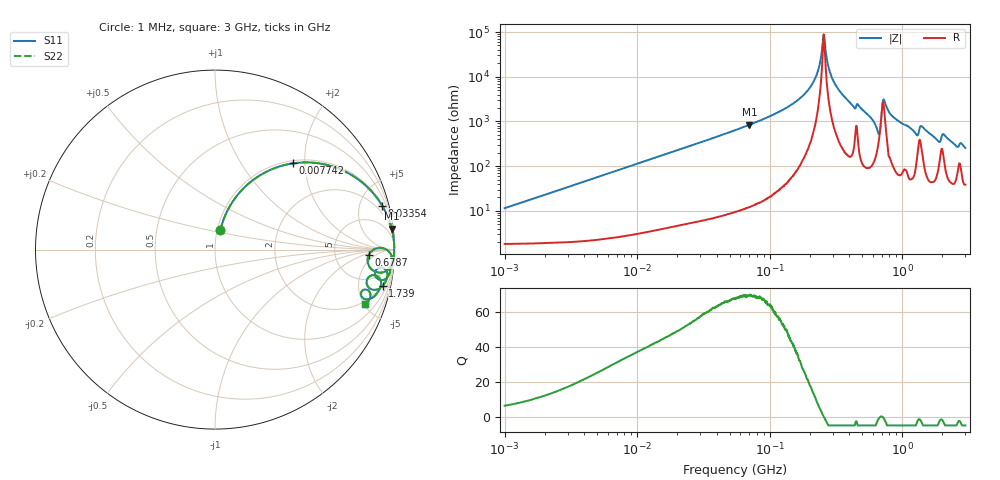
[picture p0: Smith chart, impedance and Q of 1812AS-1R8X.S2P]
!s-Parameter Generated by FASTRON Sdn. Bhd.
!FASTRON P/N : 1812AS-1R8X
!Keysight Technologies,E4991B,MY54100416,A.01.15
!Date created: Fri Oct 13 15:33:57 2023
!Version  : Rev00 Fri Oct 13 15:33:57 2023
!Data & Calibration Information:
!Freq	S11	S21	S12	S22
!PortZ  Port1:50+j0  Port2:50+j0
!When reading, reference impedance value at option line is always used.
! Remarks : This data is being provided solely for informational purposes.
# Hz S dB R 50
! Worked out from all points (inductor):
!   1601 points, 1 MHz to 3 GHz, reference 50 ohm
!   read as one part in series: L = 1.81 uH near 1.041 MHz
!   highest Q = 69.2 at 70.34 MHz (marker M1), where L = 1.9 uH
!   self-resonance near 255.8 MHz
!   S11 on the Smith chart (normalised r, x): 1 MHz: 1.04, +0.23; 7.742 MHz: 1.05, +1.74; 33.54 MHz: 1.13, +7.58; 678.7 MHz: 12, -3; 1.739 GHz: 1.90, -8.97; 3 GHz: 1.77, -5.06
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1000000  -19.00 74.5  -0.21 -6.4  -0.21 -6.4  -19.00 74.5
3804036  -8.21 64.4  -0.89 -22.8  -0.89 -22.8  -8.21 64.4
7741750  -3.77 47.9  -2.59 -40.4  -2.59 -40.4  -3.77 47.9
1.447069e7  -1.48 31.2  -5.70 -57.4  -5.70 -57.4  -1.48 31.2
3.354185e7  -0.33 14.7  -11.90 -74.3  -11.90 -74.3  -0.33 14.7
5.477226e7  -0.13 8.9  -16.19 -80.2  -16.19 -80.2  -0.13 8.9
7.034296e7  -0.08 6.8  -18.57 -82.4  -18.57 -82.4  -0.08 6.8
1.445978e8  -0.02 2.5  -27.34 -86.2  -27.34 -86.2  -0.02 2.5
2.083556e8  -0.01 0.9  -36.47 -85.4  -36.47 -85.4  -0.01 0.9
2.302869e8  -0.01 0.4  -42.20 -81.8  -42.20 -81.8  -0.01 0.4
2.570867e8  -0.01 -0.0  -58.66 12.9  -58.66 12.9  -0.01 -0.0
2.870054e8  -0.01 -0.5  -41.52 81.4  -41.52 81.4  -0.01 -0.5
3.301716e8  -0.01 -1.1  -34.35 84.8  -34.35 84.8  -0.01 -1.1
6.520712e8  -0.62 -7.9  -16.49 58.9  -16.49 58.9  -0.62 -7.9
6.787043e8  -1.34 -2.0  -16.66 11.8  -16.66 11.8  -1.34 -2.0
7.279565e8  -0.20 -1.3  -29.94 44.9  -29.94 44.9  -0.20 -1.3
7.925923e8  -0.07 -3.4  -24.41 80.8  -24.41 80.8  -0.07 -3.4
1.262285e9  -0.40 -10.1  -14.97 70.5  -14.97 70.5  -0.40 -10.1
1.409185e9  -0.36 -6.9  -18.12 67.4  -18.12 67.4  -0.36 -6.9
1.738771e9  -0.39 -12.2  -13.47 72.1  -13.47 72.1  -0.39 -12.2
2.071593e9  -0.57 -10.3  -14.65 64.9  -14.65 64.9  -0.57 -10.3
3e9  -1.04 -20.1  -9.20 61.3  -9.20 61.3  -1.04 -20.1
